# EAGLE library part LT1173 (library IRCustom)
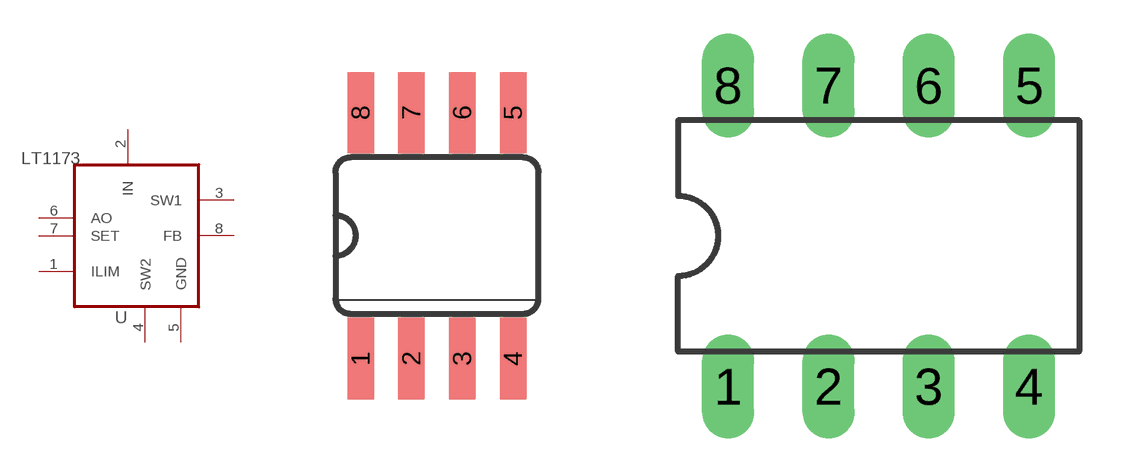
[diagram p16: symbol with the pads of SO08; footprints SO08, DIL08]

Designator prefix -

## LT1173CS  [SO08]
1  ILIM  pas
2  IN  in
3  SW1  pas
4  SW2  pas
5  GND  pwr
6  AO  out
7  SET  in
8  FB  sup

## LT1173CN  [DIL08]
Pads as for SO08

## Footprint SO08 (pad centres in mm)
smd 0.66 x 2.032: 1 -1.905,-3.073; 2 -0.635,-3.073; 3 0.635,-3.073; 4 1.905,-3.073; 5 1.905,3.073; 6 0.635,3.073; 7 -0.635,3.073; 8 -1.905,3.073

## Footprint DIL08 (pad centres in mm)
Dual In Line Package
drill 0.813 long: 1 -3.81,-3.81; 2 -1.27,-3.81; 3 1.27,-3.81; 4 3.81,-3.81; 5 3.81,3.81; 6 1.27,3.81; 7 -1.27,3.81; 8 -3.81,3.81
